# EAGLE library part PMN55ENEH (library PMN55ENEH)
MOSFET 60 V, N-channel Trench MOSFET Source: Datasheet
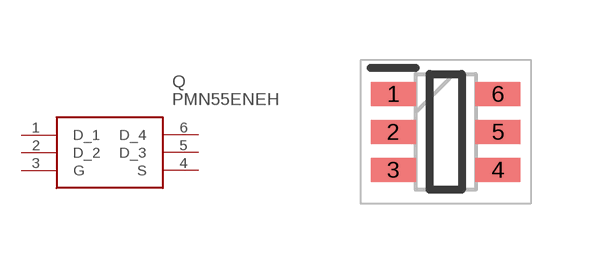
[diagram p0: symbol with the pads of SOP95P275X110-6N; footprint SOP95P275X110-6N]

Designator prefix Q

## PMN55ENEH (Arrow_Part_Number: PMN55ENEH; Arrow_Price-Stock: https://www.arrow.com/en/products/pmn55eneh/nexperia; Description: MOSFET 60 V, N-channel Trench MOSFET; Height: 1.1mm; Manufacturer_Name: Nexperia; Manufacturer_Part_Number: PMN55ENEH; Mouser_Part_Number: 771-PMN55ENEH; Mouser_Price-Stock: https://www.mouser.co.uk/ProductDetail/Nexperia/PMN55ENEH?qs=vLWxofP3U2wt3EbnGqgLRw%3D%3D)  [SOP95P275X110-6N]
1  D_1  in
2  D_2  in
3  G  in
4  S
5  D_3  in
6  D_4  in

## Footprint SOP95P275X110-6N (pad centres in mm)
TSOP-6 (SOT457)
smd 1.125 x 0.6: 1 -1.312,0.95; 2 -1.312,0; 3 -1.312,-0.95; 4 1.312,-0.95; 5 1.312,0; 6 1.312,0.95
